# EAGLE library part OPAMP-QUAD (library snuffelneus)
Operational Amplifier
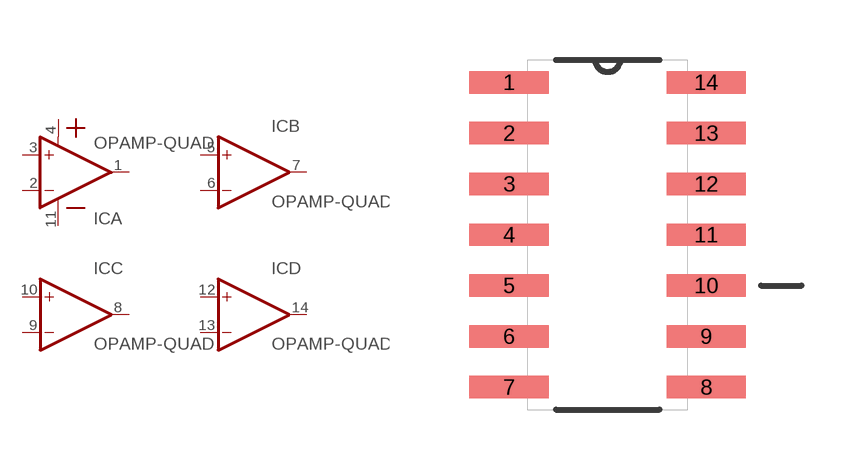
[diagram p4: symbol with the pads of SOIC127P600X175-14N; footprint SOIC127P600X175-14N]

Designator prefix IC; gates A=OP-AMP+- B=OP-AMP C=OP-AMP D=OP-AMP

## OPAMP-QUAD  [SOIC127P600X175-14N]
1  A:OUT  out
2  A:-IN  in
3  A:+IN  in
4  A:VDD  pwr
5  B:+IN  in
6  B:-IN  in
7  B:OUT  out
8  C:OUT  out
9  C:-IN  in
10  C:+IN  in
11  A:GND  pwr
12  D:+IN  in
13  D:-IN  in
14  D:OUT  out

## Footprint SOIC127P600X175-14N (pad centres in mm)
smd 1.981 x 0.559: 1 -2.464,3.81; 2 -2.464,2.54; 3 -2.464,1.27; 4 -2.464,0; 5 -2.464,-1.27; 6 -2.464,-2.54; 7 -2.464,-3.81; 8 2.464,-3.81; 9 2.464,-2.54; 10 2.464,-1.27; 11 2.464,0; 12 2.464,1.27; 13 2.464,2.54; 14 2.464,3.81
